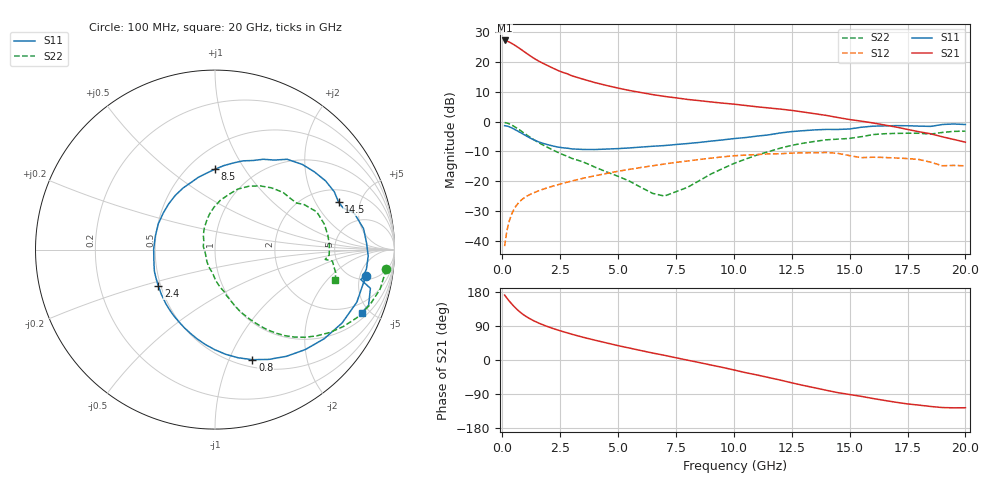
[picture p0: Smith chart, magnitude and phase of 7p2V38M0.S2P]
! Infineon Technologies  Discrete & RF Semiconductors
! bfp620
! VCE =  2.3 V,  IC =  8.0 mA
! Common Emitter S-Parameters:  Sep 2002
# GHz  S  MA  R  50
!  f  S11  S21  S12  S22
! GHz  MAG  ANG  MAG  ANG  MAG  ANG  MAG  ANG
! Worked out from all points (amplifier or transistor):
!   59 points, 100 MHz to 20 GHz, reference 50 ohm
!   highest |S21| = 27.1 dB at 100 MHz (marker M1)
!   |S21| within 3 dB of that: start of sweep to 810 MHz
!   unconditionally stable (mu >= 1): 4.193 GHz to 11.11 GHz; 17.14 GHz to end of sweep
!   at 1 GHz: K = 0.45, MSG = 24.1 dB, |S12| = -25.2 dB
!   at 5.5 GHz: K = 1.05, MAG = 11.8 dB, |S12| = -16.0 dB
!   at 20 GHz: K = 1.30, MAG = 0.7 dB, |S12| = -14.8 dB
!   S11 on the Smith chart (normalised r, x): 100 MHz: 5.73, -6.23; 800 MHz: 0.58, -1.22; 2.4 GHz: 0.48, -0.23; 8.5 GHz: 0.66, +0.74; 14.5 GHz: 2.73, +3.17; 20 GHz: 1.33, -4.50
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0.1  0.8529 -10.0  22.57 171.4  0.0083 64.6  0.9607 -6.5
0.2  0.8428 -20.3  22.05 163.2  0.0151 72.0  0.9458 -13.5
0.3  0.8177 -30.0  21.22 155.6  0.0219 70.5  0.9155 -19.8
0.4  0.7854 -39.2  20.23 148.5  0.0282 67.5  0.8765 -25.7
0.5  0.7506 -47.9  19.18 141.8  0.034 64.3  0.8331 -31.0
0.6  0.7155 -56.2  18.13 135.6  0.0393 61.3  0.788 -35.9
0.8  0.6479 -71.2  16.07 124.8  0.048 56.1  0.6994 -44.3
0.9  0.616 -78.0  15.11 120.1  0.0517 54.0  0.6575 -47.8
1.1  0.5573 -90.2  13.33 112.1  0.0579 50.5  0.5809 -53.5
1.4  0.4869 -106.2  11.17 102.3  0.0656 46.8  0.4871 -59.8
1.6  0.4532 -115.6  10.07 96.8  0.0704 45.1  0.4381 -63.1
1.9  0.4169 -128.3  8.805 89.4  0.0772 43.1  0.38 -67.2
2.4  0.3749 -147.5  7.135 79.0  0.0881 40.3  0.3055 -72.3
3.5  0.3417 179.6  5.078 59.8  0.1132 34.0  0.211 -82.3
5  0.353 144.9  3.614 37.9  0.1476 24.1  0.1219 -99.4
7  0.3967 109.8  2.63 12.4  0.1951 8.8  0.057 -165.6
8.5  0.4473 90.2  2.232 -6.6  0.2321 -4.7  0.1025 129.4
10.5  0.5401 66.8  1.853 -33.3  0.2751 -26.7  0.2354 91.5
13.5  0.7252 31.9  1.349 -73.4  0.3015 -59.5  0.4661 47.6
14.5  0.7376 21.0  1.165 -86.2  0.2942 -74.2  0.508 34.1
17  0.8544 -2.5  0.81 -111.5  0.2461 -90.6  0.6337 7.4
20  0.8905 -23.2  0.452 -126.0  0.1822 -102.7  0.691 -14.3
